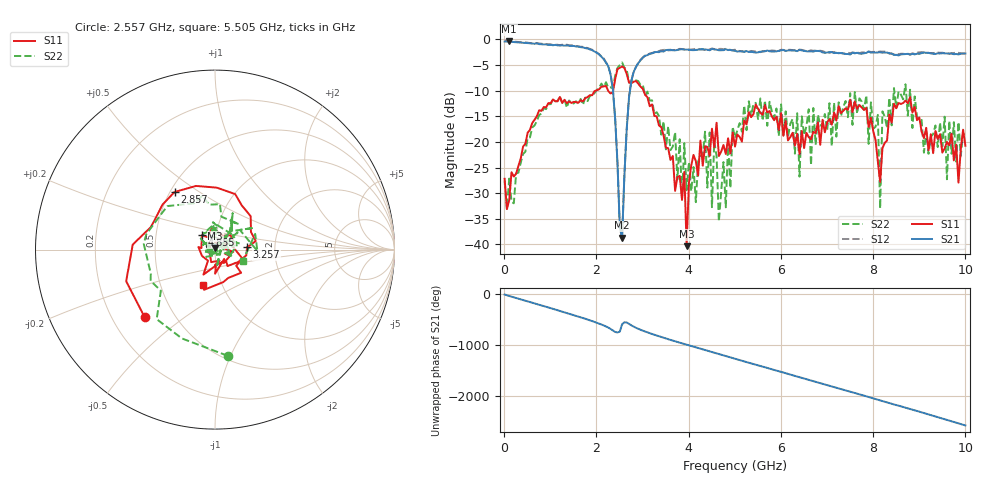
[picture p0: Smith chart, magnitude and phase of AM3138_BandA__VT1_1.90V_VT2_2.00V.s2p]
! Date/Time: Tue, Nov 13, 2018 4:42 PM
! Network Analyzer: Agilent Technologies E8364B Rev: A.07.50.67
! Sweep from 0.010 to 10.000 GHz, 201 Points, Sweep Type: LIN
! Power Supply: 1.900 V, 0.000 A
# Hz S DB R 50
!freq MagS11 AngS11 MagS21 AngS21 MagS12 AngS12 MagS22 AngS22
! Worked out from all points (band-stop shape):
!   201 points, 10 MHz to 10 GHz, reference 50 ohm
!   highest |S21| = -0.39 dB at 109.9 MHz (marker M1); lowest = -38.7 dB at 2.557 GHz (marker M2)
!   |S21| within 3 dB of the highest: start of sweep to 2.11 GHz; 3.033 GHz to end of sweep
!   lowest |S11| = -40.3 dB at 3.956 GHz (marker M3), VSWR 1.02, Z = 50.1 + j0.956 ohm
!   |S11| at or under -10 dB: start of sweep to 1.988 GHz; 2.253 GHz to 2.364 GHz (111 MHz wide, 4.81 % of centre); 3.022 GHz to end of sweep
!   |S22| runs from -35.5 to -4.5 dB; largest |S21 - S12| = 0.03
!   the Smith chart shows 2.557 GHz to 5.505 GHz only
!   S11 on the Smith chart (normalised r, x): 2.557 GHz: 0.34, -0.36; 2.857 GHz: 0.53, +0.40; 3.257 GHz: 1.43, +0.04; 4.855 GHz: 0.85, +0.14; 5.505 GHz: 0.81, -0.34
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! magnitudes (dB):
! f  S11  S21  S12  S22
! 10 MHz  -27.2  -0.4  -0.2  -27.7
! 109.9 MHz  -31.4  -0.4  -0.3  -27.2
! 1.708 GHz  -12.1  -1.6  -1.5  -12.8
! 2.308 GHz  -10.6  -6.9  -6.8  -9.4
! 2.557 GHz  -5.3  -38.7  -38.6  -4.5
! 2.857 GHz  -8.1  -5.4  -5.4  -8.0
! 3.257 GHz  -14.9  -2.5  -2.6  -14.6
! 3.357 GHz  -16.8  -2.5  -2.3  -15.0
! 3.956 GHz  -40.3  -2.0  -2.0  -29.4
! 4.106 GHz  -22.5  -2.1  -1.9  -24.9
! 4.555 GHz  -21.1  -2.0  -1.9  -19.9
! 4.655 GHz  -22.7  -2.1  -1.9  -35.5
! 4.855 GHz  -19.3  -2.1  -2.0  -19.9
! 5.005 GHz  -20.9  -2.2  -2.0  -19.2
! 5.505 GHz  -13.5  -2.5  -2.4  -15.5
! 6.703 GHz  -18.0  -2.4  -2.2  -13.4
! 7.852 GHz  -13.3  -2.6  -2.6  -10.9
! 8.102 GHz  -23.8  -2.6  -2.5  -14.7
! 8.152 GHz  -27.8  -2.5  -2.4  -33.0
! 8.202 GHz  -21.2  -2.6  -2.4  -14.0
! 8.352 GHz  -14.7  -2.7  -2.8  -11.4
! 10 GHz  -20.7  -2.8  -2.7  -19.1
